(* Logix 5000 Program export IO_Mapping; software revision 30.00 *)

TYPE Std_DiscreteAlarm :   // ALARM RESET
STRUCT
   AckC : BOOL;   // ALARM ACKNOWLEDGE
   LatchA : BOOL;   // ALARM LATCH
   DetectS : BOOL;   // ALARM DETECT
   BitS : BOOL;   // ALARM MISCOMPARE
   InhibitC : BOOL;   // ALARM INHIBIT
   Tmr : TIMER;   // ALARM Timer
END_STRUCT
END_TYPE

TYPE VMAC_DATA_INTERNAL :
STRUCT
   VMACOK : BOOL;
   CommsOK : BOOL;
   KeyOK : BOOL;
   KsInUse : BOOL;
   KsPrimeInUse : BOOL;
   EntryStatus : INT;
   NodeID : DINT;
   DestinationID : DINT;
   Counter : LINT;
   LastCounter : LINT;
   KeyID : LINT;
   VMAC_KEY : DINT[8];
   VMAC_CALC : DINT[8];
   VMAC_INPUT : DINT[8];
   DATA_INPUT : DINT[1600];
   DATA_VERIFIED : DINT[1600];
   VMAC_CTRL : VMAC;
   KeyAlarm : Std_DiscreteAlarm;
   ReplayAlarm : Std_DiscreteAlarm;
   InvalidAlarm : Std_DiscreteAlarm;
   NodeAlarm : Std_DiscreteAlarm;
   DestinationAlarm : Std_DiscreteAlarm;
   L_LES : L_LES;
   L_EQU : L_EQU;
   CommsTimer : TIMER;
END_STRUCT
END_TYPE

TYPE VMAC_DATA_MSG :
STRUCT
   STATUS : CONNECTION_STATUS;
   DATA : DINT[100];
   LEN : DINT;
   ROUNDS : DINT;
   VMAC : DINT[8];
END_STRUCT
END_TYPE

ADD_ON_INSTRUCTION D_SHR   (* revision 1.0 20170524, vendor Kenneth A. Fischer *)
// DINT bit shift right of the 32-bit argument Inp_A by Inp_B bits with paddding by zeros on the right
// Revision note:
// Rev1.0: 20170524 - Initial Release
VAR_IN_OUT
   Inp_A : DINT; {required}   // 64-bit Integer to be right circular rotated
END_VAR
VAR_INPUT
   Inp_B : INT; {required}   // Number of bits to shift
END_VAR
VAR_IN_OUT
   Out : DINT; {required}   // Result
END_VAR
VAR
   BSR_Cntrl : CONTROL := (LEN := 32);
   ONS : BOOL;
   Source_Bit : BOOL;
   Wrk_InpA : DINT[2];
END_VAR

ROUTINE Logic   (* ladder *)
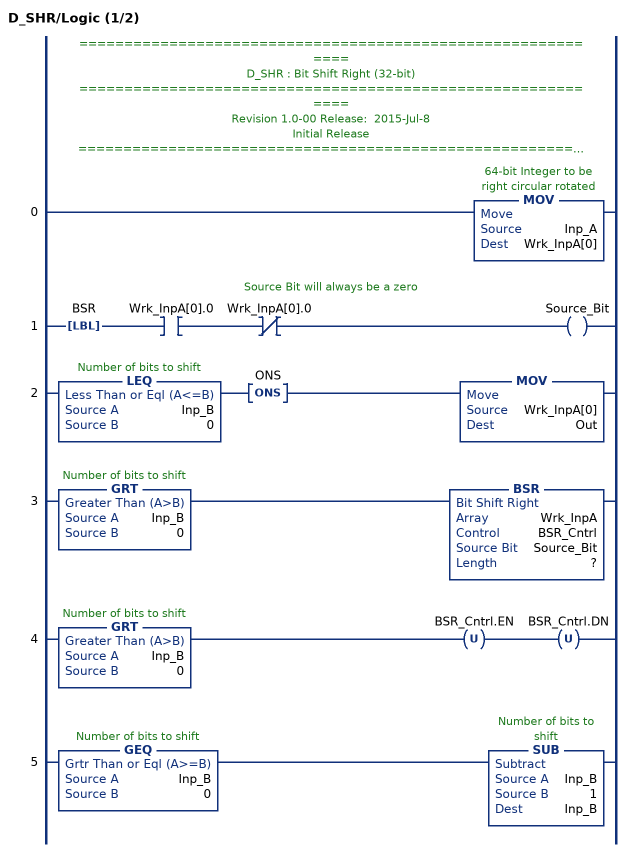
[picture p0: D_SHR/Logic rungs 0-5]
   // ============================================================
   // D_SHR : Bit Shift Right (32-bit)
   // ============================================================
   // Revision 1.0-00 Release:  2015-Jul-8
   // Initial Release
   // ============================================================
   // Performs a right bit shift of the 32-bit argument Inp_A by the
   // number of bits defined in the 16-bit argument Inp_B, with padding by zeros.
   0: MOV(Inp_A,Wrk_InpA[0]);
   // Source Bit will always be a zero
   1: LBL(BSR)XIC(Wrk_InpA[0].0)XIO(Wrk_InpA[0].0)OTE(Source_Bit);
   2: LEQ(Inp_B,0)ONS(ONS)MOV(Wrk_InpA[0],Out);
   3: GRT(Inp_B,0)BSR(Wrk_InpA,BSR_Cntrl,Source_Bit,?);
   4: GRT(Inp_B,0)OTU(BSR_Cntrl.EN)OTU(BSR_Cntrl.DN);
   5: GEQ(Inp_B,0)SUB(Inp_B,1,Inp_B);
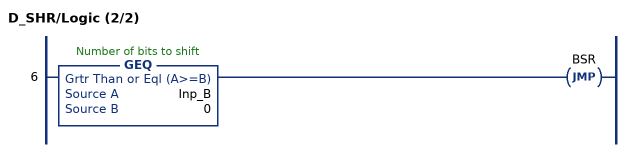
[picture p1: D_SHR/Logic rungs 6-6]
   6: GEQ(Inp_B,0)JMP(BSR);
END_ROUTINE
END_ADD_ON_INSTRUCTION

ADD_ON_INSTRUCTION D_SHL   (* revision 1.0 20170524, vendor Kenneth A. Fischer *)
// DINT bit shift left of the 32-bit argument Inp_A by Inp_B bits with paddding by zeros on the right
// Revision note:
// Rev1.0: 20170524 - Initial Release
VAR_IN_OUT
   Inp_A : DINT; {required}   // 64-bit Integer to be right circular rotated
END_VAR
VAR_INPUT
   Inp_B : INT; {required}   // Number of bits to shift
END_VAR
VAR_IN_OUT
   Out : DINT; {required}   // Result
END_VAR
VAR
   Wrk_InpA : DINT[2];
   Source_Bit : BOOL;
   ONS : BOOL;
   BSL_Cntrl : CONTROL := (LEN := 32);
END_VAR

ROUTINE Logic   (* ladder *)
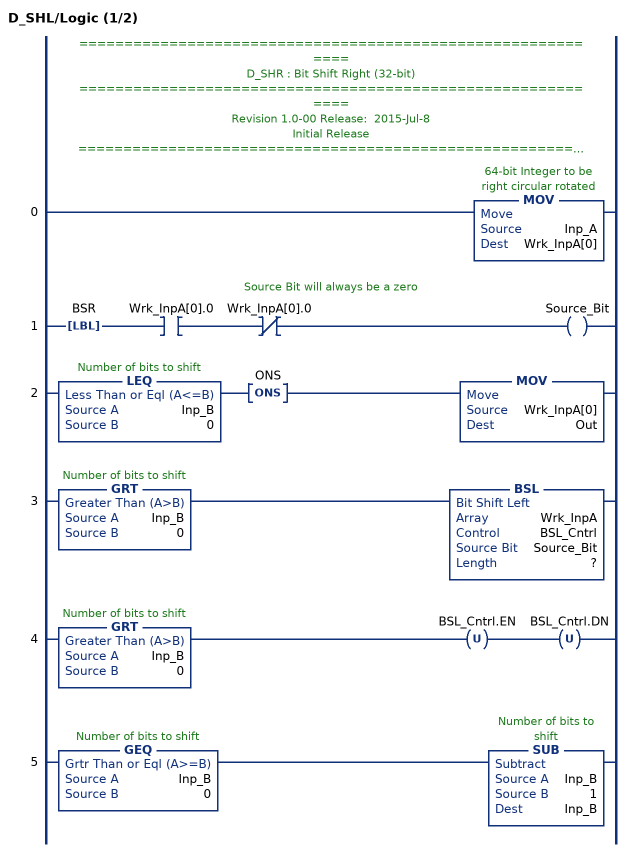
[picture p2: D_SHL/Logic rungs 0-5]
   // ============================================================
   // D_SHR : Bit Shift Right (32-bit)
   // ============================================================
   // Revision 1.0-00 Release:  2015-Jul-8
   // Initial Release
   // ============================================================
   // Performs a left bit shift of the 32-bit argument Inp_A by the
   // number of bits defined in the 16-bit argument Inp_B, with padding by zeros.
   0: MOV(Inp_A,Wrk_InpA[0]);
   // Source Bit will always be a zero
   1: LBL(BSR)XIC(Wrk_InpA[0].0)XIO(Wrk_InpA[0].0)OTE(Source_Bit);
   2: LEQ(Inp_B,0)ONS(ONS)MOV(Wrk_InpA[0],Out);
   3: GRT(Inp_B,0)BSL(Wrk_InpA,BSL_Cntrl,Source_Bit,?);
   4: GRT(Inp_B,0)OTU(BSL_Cntrl.EN)OTU(BSL_Cntrl.DN);
   5: GEQ(Inp_B,0)SUB(Inp_B,1,Inp_B);
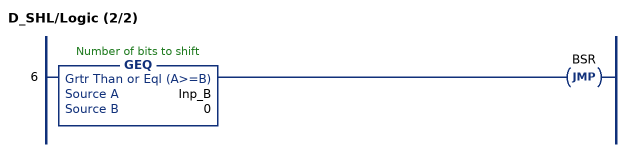
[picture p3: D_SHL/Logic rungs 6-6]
   6: GEQ(Inp_B,0)JMP(BSR);
END_ROUTINE
END_ADD_ON_INSTRUCTION

ADD_ON_INSTRUCTION B256_CtoE   (* revision 1.0 20170916, vendor Kenneth A. Fischer *)
// Convert 256-bit value using 22 12-bit pieces into 256-bit value using 32 8-bit pieces
// Revision note:
// Rev1.0: 20170916 - Initial Release
VAR_IN_OUT
   Inp_C : DINT[22]; {required}
   Out_E : DINT[32]; {required}
END_VAR
VAR
   i : INT;
   j : INT;
   TEMP1 : DINT;
   TEMP2 : DINT;
   D_SHL : D_SHL;
   D_SHR : D_SHR;
END_VAR

ROUTINE Logic   (* ladder *)
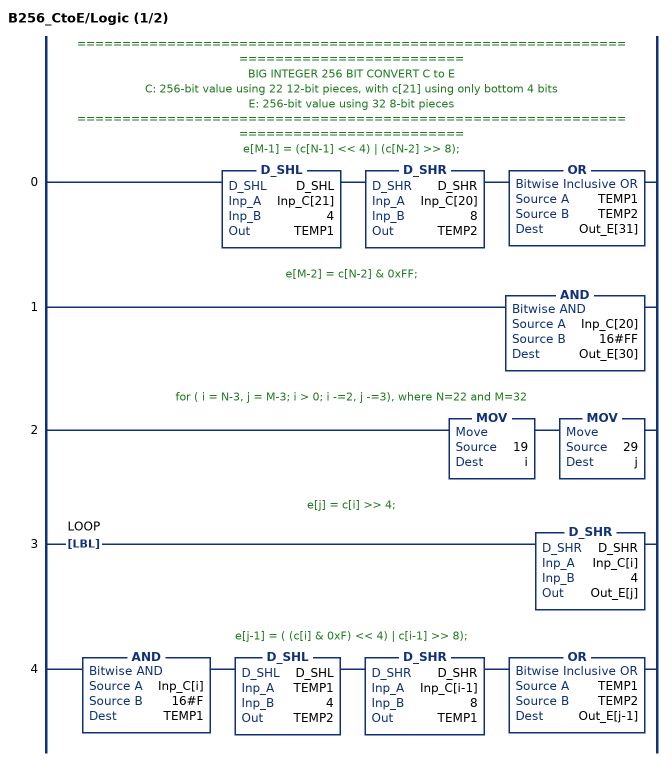
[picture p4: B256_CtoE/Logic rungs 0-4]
   // ======================================================================================
   // BIG INTEGER 256 BIT CONVERT C to E
   // C: 256-bit value using 22 12-bit pieces, with c[21] using only bottom 4 bits
   // E: 256-bit value using 32 8-bit pieces
   // ======================================================================================
   // e[M-1] = (c[N-1] << 4) | (c[N-2] >> 8);
   0: D_SHL(D_SHL,Inp_C[21],4,TEMP1)D_SHR(D_SHR,Inp_C[20],8,TEMP2)OR(TEMP1,TEMP2,Out_E[31]);
   // e[M-2] = c[N-2] & 0xFF;
   1: AND(Inp_C[20],16#FF,Out_E[30]);
   // for ( i = N-3, j = M-3; i > 0; i -=2, j -=3), where N=22 and M=32
   2: MOV(19,i)MOV(29,j);
   // e[j] = c[i] >> 4;
   3: LBL(LOOP)D_SHR(D_SHR,Inp_C[i],4,Out_E[j]);
   // e[j-1] = ( (c[i] & 0xF) << 4) | c[i-1] >> 8);
   4: AND(Inp_C[i],16#F,TEMP1)D_SHL(D_SHL,TEMP1,4,TEMP2)D_SHR(D_SHR,Inp_C[i-1],8,TEMP1)OR(TEMP1,TEMP2,Out_E[j-1]);
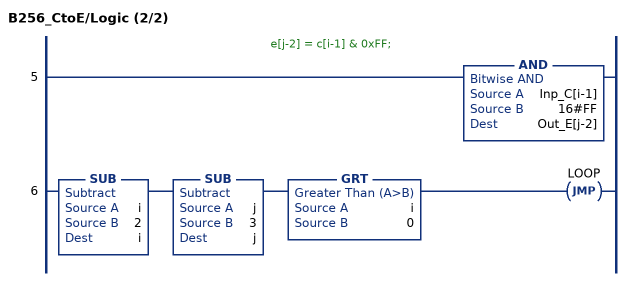
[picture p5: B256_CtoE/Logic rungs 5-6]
   // e[j-2] = c[i-1] & 0xFF;
   5: AND(Inp_C[i-1],16#FF,Out_E[j-2]);
   6: SUB(i,2,i)SUB(j,3,j)GRT(i,0)JMP(LOOP);
END_ROUTINE
END_ADD_ON_INSTRUCTION

ADD_ON_INSTRUCTION B256_StoC   (* revision 1.0 20170916, vendor Kenneth A. Fischer *)
// Convert 256-bit value using 64 hex string characters into 256-bit value using 22 12-bit pieces
// Revision note:
// Rev1.0: 20170916 - Initial Release
VAR_IN_OUT
   Inp_S : STRING; {required}
   Out_C : DINT[22]; {required}
END_VAR
VAR
   byte : DINT[3];
   D_SHL : D_SHL;
   i : INT;
   j : INT;
   k : DINT;
   temp : DINT;
END_VAR

ROUTINE Logic   (* ladder *)
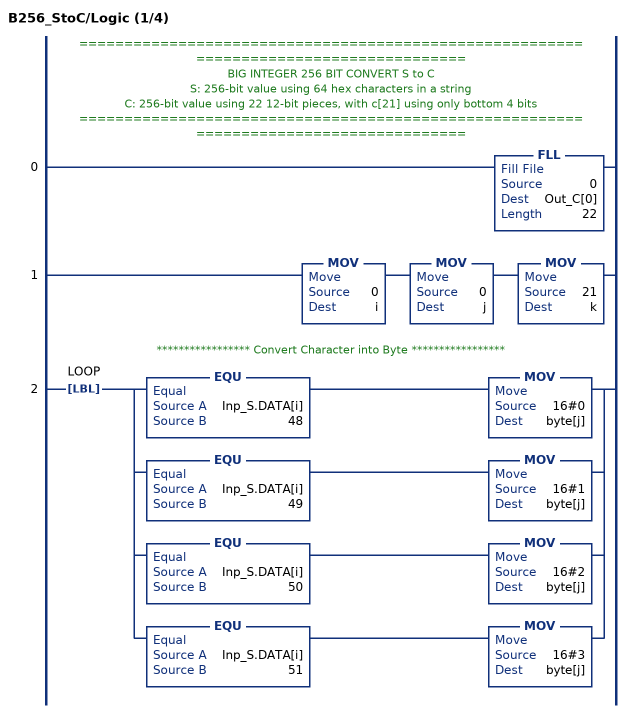
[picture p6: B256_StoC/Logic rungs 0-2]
   // ======================================================================================
   // BIG INTEGER 256 BIT CONVERT S to C
   // S: 256-bit value using 64 hex characters in a string
   // C: 256-bit value using 22 12-bit pieces, with c[21] using only bottom 4 bits
   // ======================================================================================
   0: FLL(0,Out_C[0],22);
   1: MOV(0,i)MOV(0,j)MOV(21,k);
   // ***************** Convert Character into Byte *****************
   2: LBL(LOOP)[EQU(Inp_S.DATA[i],48) MOV(16#0,byte[j]) ,EQU(Inp_S.DATA[i],49) MOV(16#1,byte[j]) ,EQU(Inp_S.DATA[i],50) MOV(16#2,byte[j]) ,EQU(Inp_S.DATA[i],51) MOV(16#3,byte[j]) ];
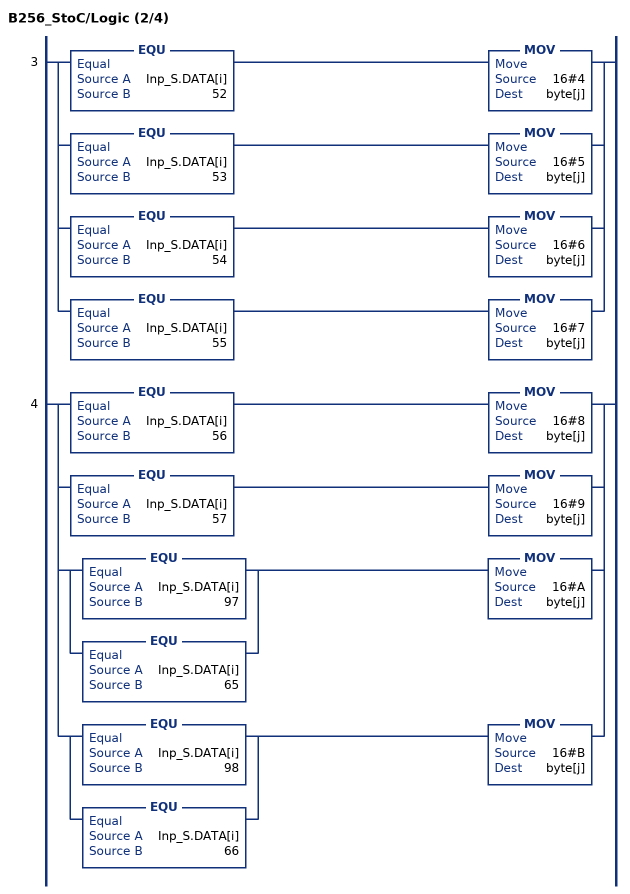
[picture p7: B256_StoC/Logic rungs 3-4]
   3: [EQU(Inp_S.DATA[i],52) MOV(16#4,byte[j]) ,EQU(Inp_S.DATA[i],53) MOV(16#5,byte[j]) ,EQU(Inp_S.DATA[i],54) MOV(16#6,byte[j]) ,EQU(Inp_S.DATA[i],55) MOV(16#7,byte[j]) ];
   4: [EQU(Inp_S.DATA[i],56) MOV(16#8,byte[j]) ,EQU(Inp_S.DATA[i],57) MOV(16#9,byte[j]) ,[EQU(Inp_S.DATA[i],97) ,EQU(Inp_S.DATA[i],65) ] MOV(16#A,byte[j]) ,[EQU(Inp_S.DATA[i],98) ,EQU(Inp_S.DATA[i],66) ] MOV(16#B,byte[j]) ];
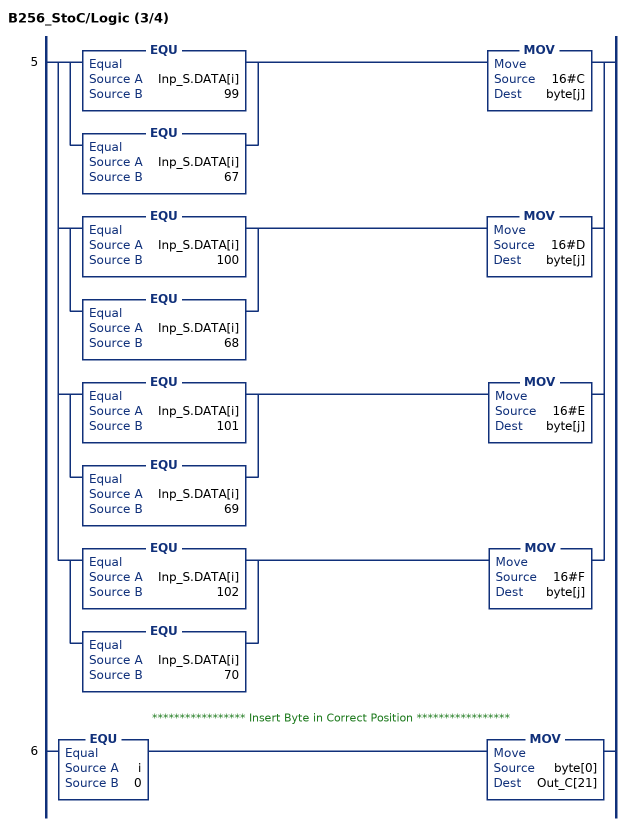
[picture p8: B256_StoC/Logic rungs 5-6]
   5: [[EQU(Inp_S.DATA[i],99) ,EQU(Inp_S.DATA[i],67) ] MOV(16#C,byte[j]) ,[EQU(Inp_S.DATA[i],100) ,EQU(Inp_S.DATA[i],68) ] MOV(16#D,byte[j]) ,[EQU(Inp_S.DATA[i],101) ,EQU(Inp_S.DATA[i],69) ] MOV(16#E,byte[j]) ,[EQU(Inp_S.DATA[i],102) ,EQU(Inp_S.DATA[i],70) ] MOV(16#F,byte[j]) ];
   // ***************** Insert Byte in Correct Position *****************
   6: EQU(i,0)MOV(byte[0],Out_C[21]);
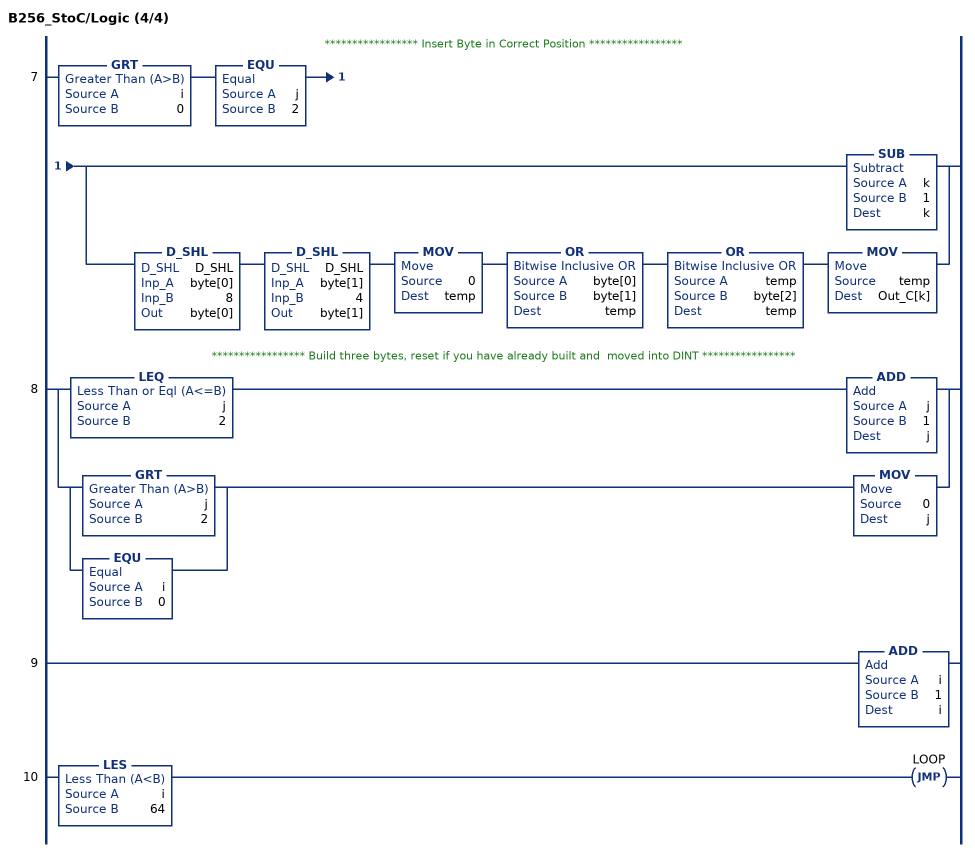
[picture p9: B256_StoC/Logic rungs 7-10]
   // ***************** Insert Byte in Correct Position *****************
   7: GRT(i,0)EQU(j,2)[SUB(k,1,k) ,D_SHL(D_SHL,byte[0],8,byte[0]) D_SHL(D_SHL,byte[1],4,byte[1]) MOV(0,temp) OR(byte[0],byte[1],temp) OR(temp,byte[2],temp) MOV(temp,Out_C[k]) ];
   // ***************** Build three bytes, reset if you have already built and  moved into DINT *****************
   8: [LEQ(j,2) ADD(j,1,j) ,[GRT(j,2) ,EQU(i,0) ] MOV(0,j) ];
   9: ADD(i,1,i);
   10: LES(i,64)JMP(LOOP);
END_ROUTINE
END_ADD_ON_INSTRUCTION

ADD_ON_INSTRUCTION L_INC   (* revision 1.0 00 Release, vendor Rockwell Automation *)
// Increment (64-bit)
// Revision note:
// Initial Release
// Help:
// This instruction increments the input 64-bit integer, returning its value plus 1.
VAR_IN_OUT
   Inp : LINT; {required}   // Input
   Out : LINT; {required}   // Output = Input + 1
END_VAR
VAR
   Wrk : DINT[2];   // Working pair of 32-bit integers (DINTs)
   Wrk_LoOvflw : BOOL;   // Low-order 32-bit overflow (without minor fault)
   Wrk_HiOvflw : BOOL;   // High-order 32-bit overflow (without minor fault)
END_VAR

ROUTINE Logic   (* ladder *)
// Output the value of the input plus 1
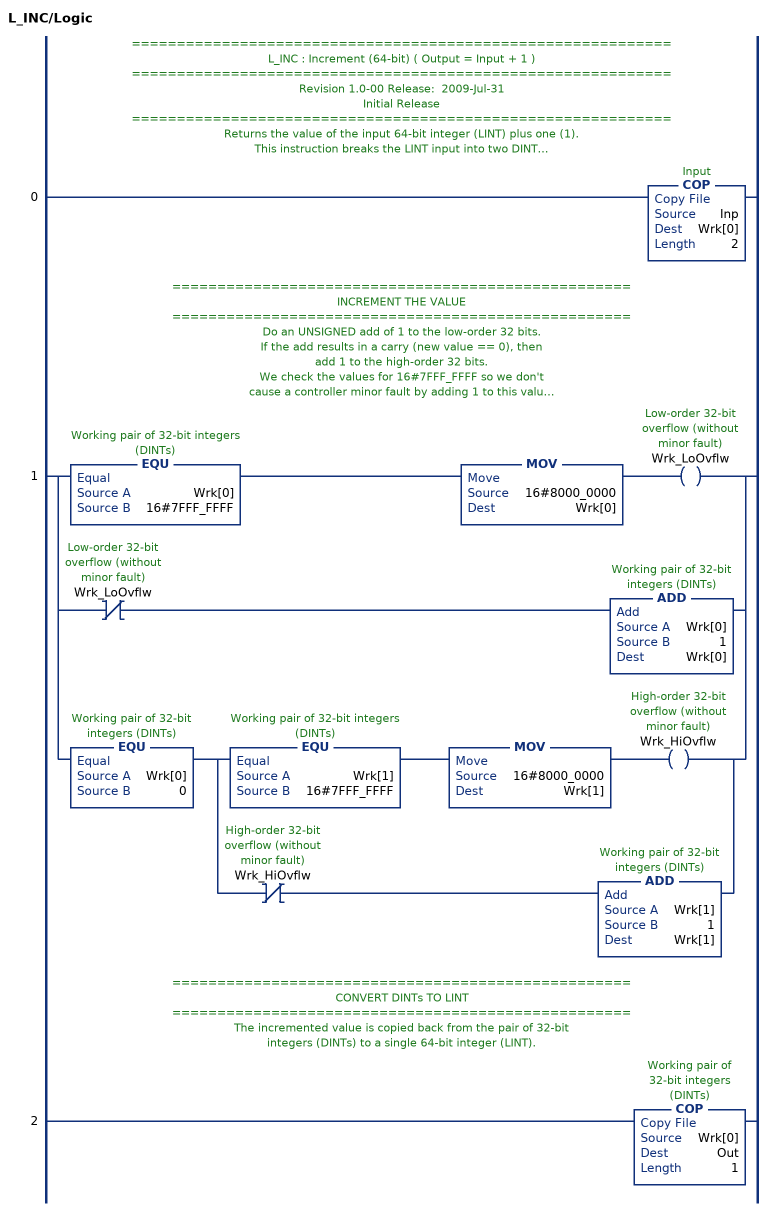
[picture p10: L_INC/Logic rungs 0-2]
   // ============================================================
   // L_INC : Increment (64-bit) ( Output = Input + 1 )
   // ============================================================
   // Revision 1.0-00 Release:  2009-Jul-31
   // Initial Release
   // ============================================================
   // Returns the value of the input 64-bit integer (LINT) plus one (1).
   // This instruction breaks the LINT input into two DINTs
   // (32-bit signed each) to do the math.
   // ===================================================
   // CONVERT LINT TO DINTs
   // ===================================================
   // This COPy takes the input LINT and breaks it into a pair of DINTs.
   0: COP(Inp,Wrk[0],2);
   // ===================================================
   // INCREMENT THE VALUE
   // ===================================================
   // Do an UNSIGNED add of 1 to the low-order 32 bits.
   // If the add results in a carry (new value == 0), then
   // add 1 to the high-order 32 bits.
   // We check the values for 16#7FFF_FFFF so we don't
   // cause a controller minor fault by adding 1 to this value
   // (resulting in a signed overflow to negative).
   1: [EQU(Wrk[0],16#7FFF_FFFF) MOV(16#8000_0000,Wrk[0]) OTE(Wrk_LoOvflw) ,XIO(Wrk_LoOvflw) ADD(Wrk[0],1,Wrk[0]) ,EQU(Wrk[0],0) [EQU(Wrk[1],16#7FFF_FFFF) MOV(16#8000_0000,Wrk[1]) OTE(Wrk_HiOvflw) ,XIO(Wrk_HiOvflw) ADD(Wrk[1],1,Wrk[1]) ] ];
   // ===================================================
   // CONVERT DINTs TO LINT
   // ===================================================
   // The incremented value is copied back from the pair of 32-bit
   // integers (DINTs) to a single 64-bit integer (LINT).
   2: COP(Wrk[0],Out,1);
END_ROUTINE
END_ADD_ON_INSTRUCTION

ADD_ON_INSTRUCTION B256_EtoDINT   (* revision 1.0 20170916, vendor Kenneth A. Fischer *)
// Convert 256-bit value using 32 8-bit pieces into 256-bit value using 8 32-bit pieces
// Revision note:
// Rev1.0: 20170916 - Initial Release
VAR_IN_OUT
   Inp_E : DINT[32]; {required}
   Out_DINT : DINT[8]; {required}
END_VAR
VAR
   D_SHL : D_SHL;
   i : INT;
   j : INT;
   TEMP : DINT;
END_VAR

ROUTINE Logic   (* ladder *)
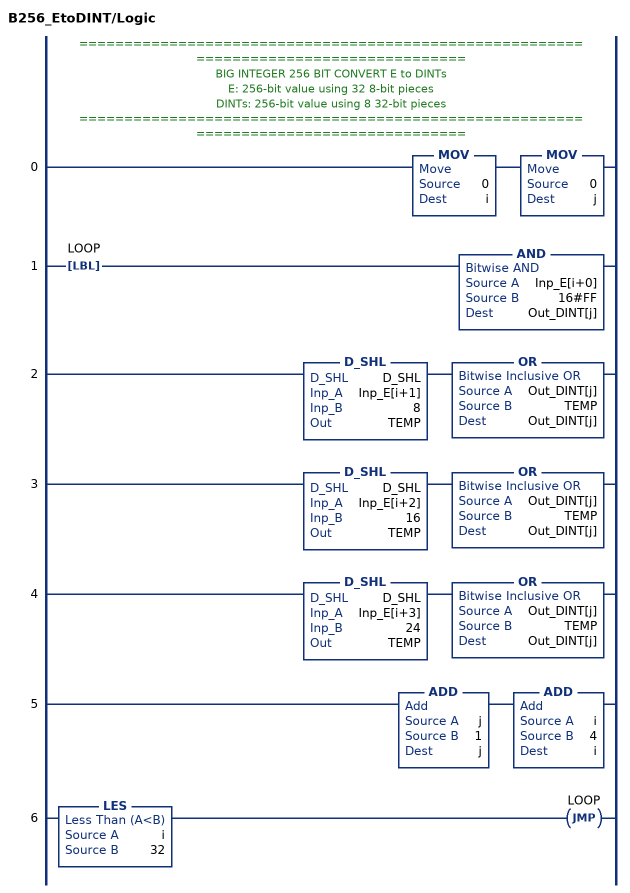
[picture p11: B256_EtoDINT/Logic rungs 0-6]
   // ======================================================================================
   // BIG INTEGER 256 BIT CONVERT E to DINTs
   // E: 256-bit value using 32 8-bit pieces
   // DINTs: 256-bit value using 8 32-bit pieces
   // ======================================================================================
   0: MOV(0,i)MOV(0,j);
   1: LBL(LOOP)AND(Inp_E[i+0],16#FF,Out_DINT[j]);
   2: D_SHL(D_SHL,Inp_E[i+1],8,TEMP)OR(Out_DINT[j],TEMP,Out_DINT[j]);
   3: D_SHL(D_SHL,Inp_E[i+2],16,TEMP)OR(Out_DINT[j],TEMP,Out_DINT[j]);
   4: D_SHL(D_SHL,Inp_E[i+3],24,TEMP)OR(Out_DINT[j],TEMP,Out_DINT[j]);
   5: ADD(j,1,j)ADD(i,4,i);
   6: LES(i,32)JMP(LOOP);
END_ROUTINE
END_ADD_ON_INSTRUCTION

ADD_ON_INSTRUCTION D_ROTR   (* revision 1.0 20170524, vendor Kenneth A. Fischer *)
// DINT circular right shift (rotation) of the 32-bit argument Inp_A by Inp_B bits
// Revision note:
// Rev1.0: 20170524 - Initial Release
VAR_IN_OUT
   Inp_A : DINT; {required}   // 64-bit Integer to be right circular rotated
END_VAR
VAR_INPUT
   Inp_B : INT; {required}   // Number of Inp_A bit rotations
END_VAR
VAR_IN_OUT
   Out : DINT; {required}   // Result
END_VAR
VAR
   Wrk_InpA : DINT[2];
   BSR_Cntrl : CONTROL := (LEN := 32);
   Source_Bit : BOOL;
   ONS : BOOL;
END_VAR

ROUTINE Logic   (* ladder *)
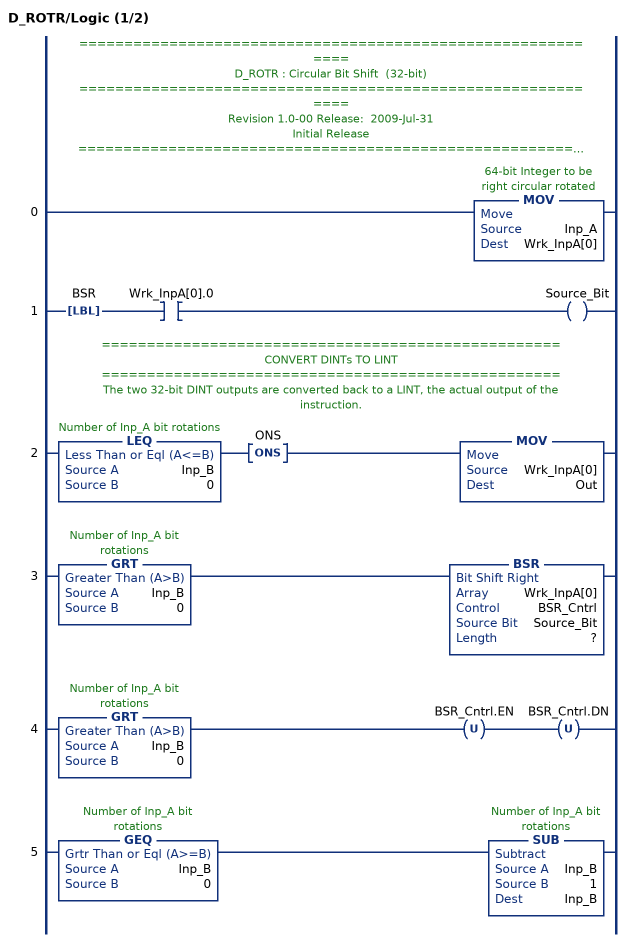
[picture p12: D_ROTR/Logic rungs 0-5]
   // ============================================================
   // D_ROTR : Circular Bit Shift  (32-bit)
   // ============================================================
   // Revision 1.0-00 Release:  2009-Jul-31
   // Initial Release
   // ============================================================
   // Performs a circular right shift rotation of the 32-bit argument Inp_A by the
   // number of bits defined in the 16-bit argument Inp_B.
   0: MOV(Inp_A,Wrk_InpA[0]);
   1: LBL(BSR)XIC(Wrk_InpA[0].0)OTE(Source_Bit);
   // ===================================================
   // CONVERT DINTs TO LINT
   // ===================================================
   // The two 32-bit DINT outputs are converted back to a LINT, the actual output of the instruction.
   2: LEQ(Inp_B,0)ONS(ONS)MOV(Wrk_InpA[0],Out);
   3: GRT(Inp_B,0)BSR(Wrk_InpA[0],BSR_Cntrl,Source_Bit,?);
   4: GRT(Inp_B,0)OTU(BSR_Cntrl.EN)OTU(BSR_Cntrl.DN);
   5: GEQ(Inp_B,0)SUB(Inp_B,1,Inp_B);
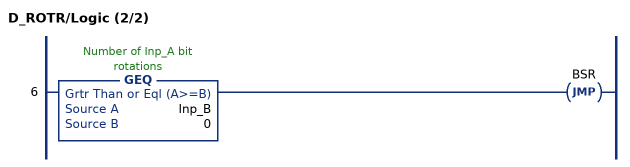
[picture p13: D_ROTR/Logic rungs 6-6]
   6: GEQ(Inp_B,0)JMP(BSR);
END_ROUTINE
END_ADD_ON_INSTRUCTION

ADD_ON_INSTRUCTION VMAC   (* revision 1.0 20170524, vendor Kenneth A. Fischer *)
// Variable Round MAC
// Revision note:
// Rev1.0: 20170524 - Initial Release
VAR_IN_OUT
   Inp_KEY : DINT[8]; {required}
   Inp_MSG : DINT[500]; {required}
END_VAR
VAR_INPUT
   Inp_LEN : DINT; {required}   // LENGTH INPUT OF MSG IN NUMBER OF DINTS
   Inp_ROUNDS : DINT; {required}
END_VAR
VAR_IN_OUT
   Out_VMAC : DINT[8]; {required}
        [0]   // HashBuffer_A
        [1]   // HashBuffer_B
        [2]   // HashBuffer_C
        [3]   // HashBuffer_D
        [4]   // HashBuffer_E
        [5]   // HashBuffer_F
        [6]   // HashBuffer_G
        [7]   // HashBuffer_H
END_VAR
VAR
   MajFunc : DINT;
   HashBuffer_H : DINT;
   HashBuffer_G : DINT;
   HashBuffer_F : DINT;
   HashBuffer_E : DINT;
   HashBuffer_D : DINT;
   HashBuffer_C : DINT;
   HashBuffer_B : DINT;
   HashBuffer_A : DINT;
   W : DINT[64];   // MESSAGE SCHEDULE
   tmp : DINT[20];
   T2 : DINT;
   T1 : DINT;
   t : INT;
   M : INT;   // MESSAGE INCREMENTS
   SigmaE : DINT;
   SigmaA : DINT;
   Sigma1 : DINT;
   Sigma0 : DINT;
   i : INT;
   x : INT;
   HashBufferInput_H : DINT;
   HashBufferInput_G : DINT;
   HashBufferInput_F : DINT;
   HashBufferInput_E : DINT;
   HashBufferInput_D : DINT;
   HashBufferInput_C : DINT;
   HashBufferInput_B : DINT;
   HashBufferInput_A : DINT;
   CondFunc : DINT;
   K : DINT[64];
   LENGTH_BITS : DINT;   // LENGTH OF MSG IN BITS
   LENGTH_MODULO : DINT;
   NUM_PADDING_BITS : DINT;   // NUMBER OF BITS NEEDED FOR PADDING
   NUM_PADDING_DINTS : DINT;   // NUMBER OF DINTS NEEDED FOR PADDING
   PADDING_COUNTER : DINT;
   TOTAL_MSG_LENGTH_MINUS_16 : DINT;
   D_ROTR : D_ROTR;
   D_SHR : D_SHR;
   ROUNDS : DINT;
   n : INT;
   KeyIndex : DINT;
   RotationIndex : DINT;
   IndexedKey : DINT;
END_VAR

ROUTINE Logic   (* ladder *)
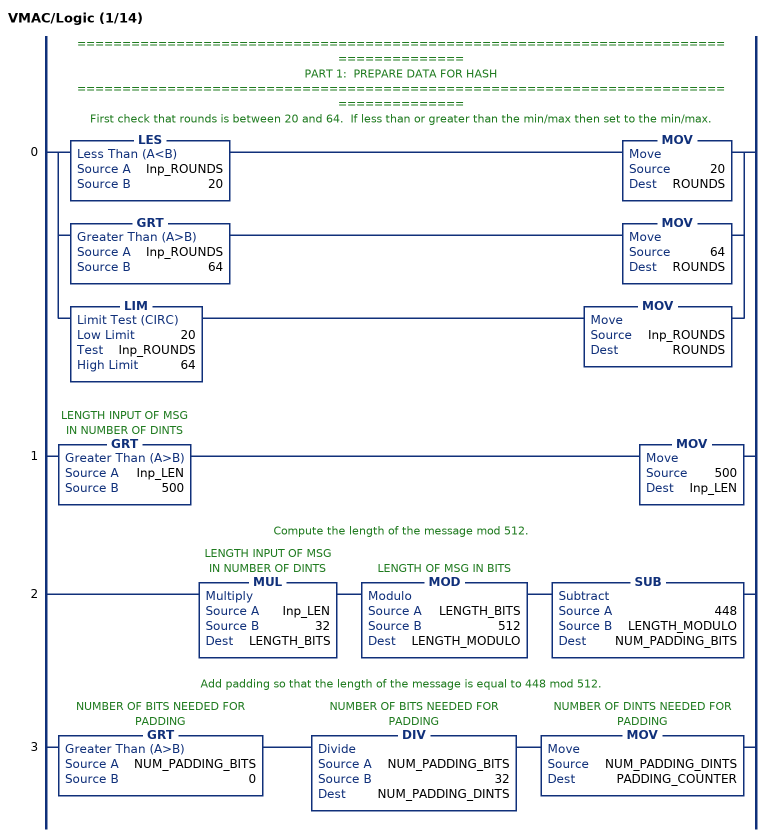
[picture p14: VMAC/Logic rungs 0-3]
   // ======================================================================================
   // PART 1:  PREPARE DATA FOR HASH
   // ======================================================================================
   // First check that rounds is between 20 and 64.  If less than or greater than the min/max then set to the min/max.
   0: [LES(Inp_ROUNDS,20) MOV(20,ROUNDS) ,GRT(Inp_ROUNDS,64) MOV(64,ROUNDS) ,LIM(20,Inp_ROUNDS,64) MOV(Inp_ROUNDS,ROUNDS) ];
   1: GRT(Inp_LEN,500)MOV(500,Inp_LEN);
   // Compute the length of the message mod 512.
   2: MUL(Inp_LEN,32,LENGTH_BITS)MOD(LENGTH_BITS,512,LENGTH_MODULO)SUB(448,LENGTH_MODULO,NUM_PADDING_BITS);
   // Add padding so that the length of the message is equal to 448 mod 512.
   3: GRT(NUM_PADDING_BITS,0)DIV(NUM_PADDING_BITS,32,NUM_PADDING_DINTS)MOV(NUM_PADDING_DINTS,PADDING_COUNTER);
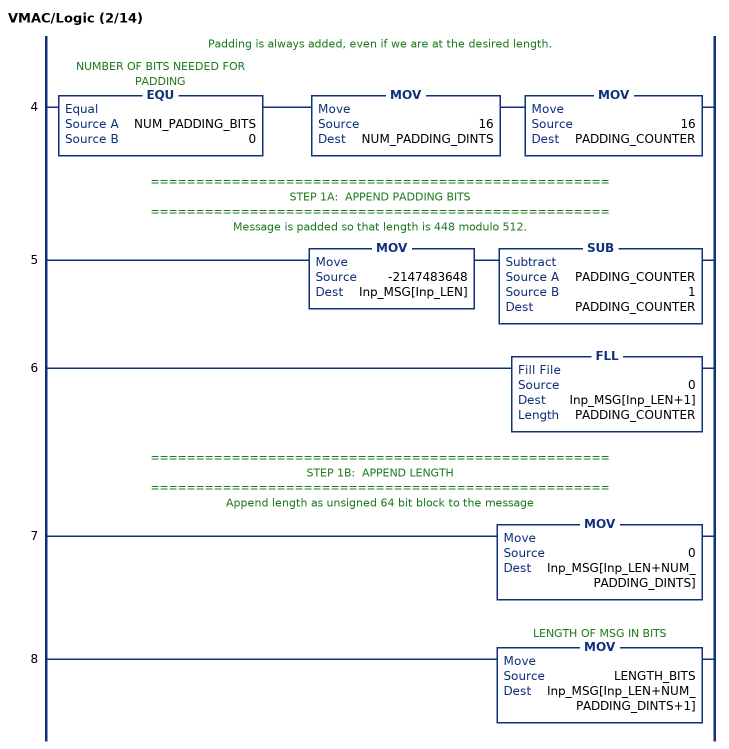
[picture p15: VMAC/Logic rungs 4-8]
   // Padding is always added, even if we are at the desired length.
   4: EQU(NUM_PADDING_BITS,0)MOV(16,NUM_PADDING_DINTS)MOV(16,PADDING_COUNTER);
   // ===================================================
   // STEP 1A:  APPEND PADDING BITS
   // ===================================================
   // Message is padded so that length is 448 modulo 512.
   5: MOV(-2147483648,Inp_MSG[Inp_LEN])SUB(PADDING_COUNTER,1,PADDING_COUNTER);
   6: FLL(0,Inp_MSG[Inp_LEN+1],PADDING_COUNTER);
   // ===================================================
   // STEP 1B:  APPEND LENGTH
   // ===================================================
   // Append length as unsigned 64 bit block to the message
   7: MOV(0,Inp_MSG[Inp_LEN+NUM_PADDING_DINTS]);
   8: MOV(LENGTH_BITS,Inp_MSG[Inp_LEN+NUM_PADDING_DINTS+1]);
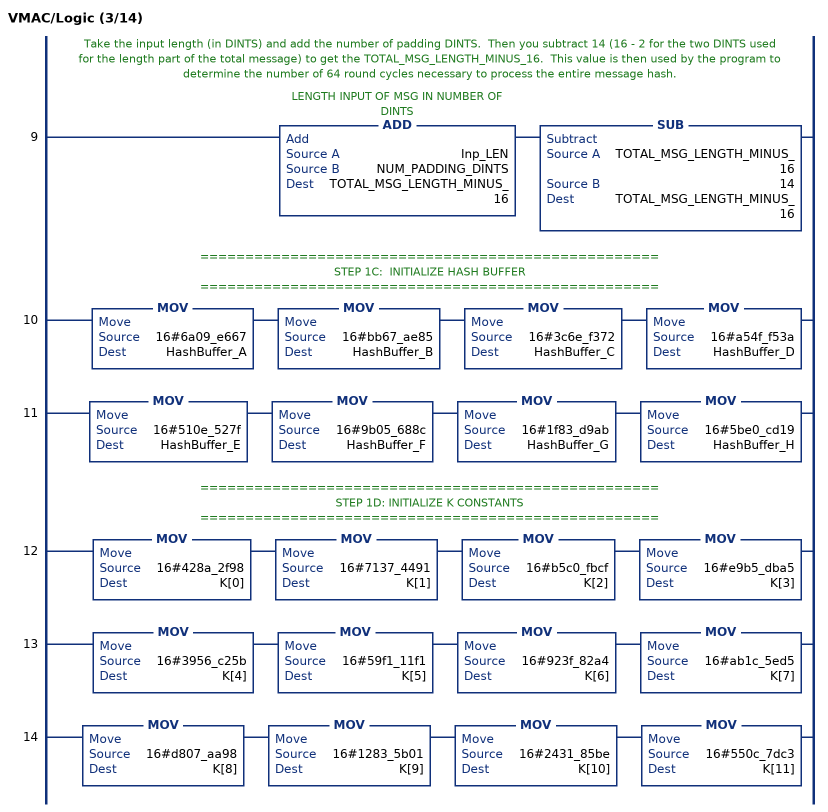
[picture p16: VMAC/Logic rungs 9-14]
   // Take the input length (in DINTS) and add the number of padding DINTS.  Then you subtract 14 (16 - 2 for the two DINTS used for the length part of the total message) to get the TOTAL_MSG_LENGTH_MINUS_16.  This value is then used by the program to determine the number of 64 round cycles necessary to process the entire message hash.
   9: ADD(Inp_LEN,NUM_PADDING_DINTS,TOTAL_MSG_LENGTH_MINUS_16)SUB(TOTAL_MSG_LENGTH_MINUS_16,14,TOTAL_MSG_LENGTH_MINUS_16);
   // ===================================================
   // STEP 1C:  INITIALIZE HASH BUFFER
   // ===================================================
   10: MOV(16#6a09_e667,HashBuffer_A)MOV(16#bb67_ae85,HashBuffer_B)MOV(16#3c6e_f372,HashBuffer_C)MOV(16#a54f_f53a,HashBuffer_D);
   11: MOV(16#510e_527f,HashBuffer_E)MOV(16#9b05_688c,HashBuffer_F)MOV(16#1f83_d9ab,HashBuffer_G)MOV(16#5be0_cd19,HashBuffer_H);
   // ===================================================
   // STEP 1D: INITIALIZE K CONSTANTS
   // ===================================================
   12: MOV(16#428a_2f98,K[0])MOV(16#7137_4491,K[1])MOV(16#b5c0_fbcf,K[2])MOV(16#e9b5_dba5,K[3]);
   13: MOV(16#3956_c25b,K[4])MOV(16#59f1_11f1,K[5])MOV(16#923f_82a4,K[6])MOV(16#ab1c_5ed5,K[7]);
   14: MOV(16#d807_aa98,K[8])MOV(16#1283_5b01,K[9])MOV(16#2431_85be,K[10])MOV(16#550c_7dc3,K[11]);
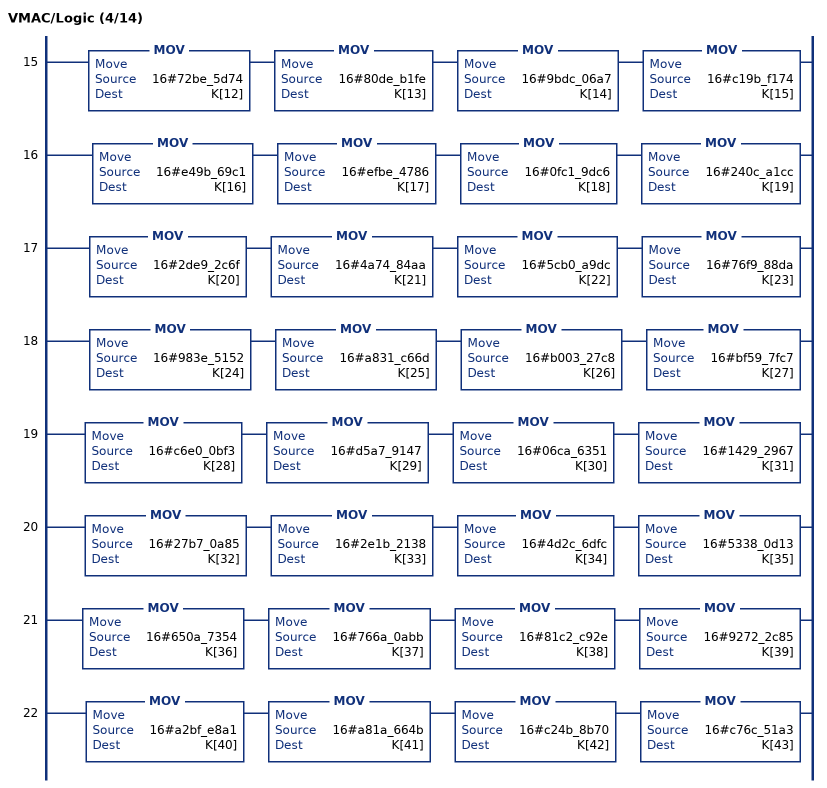
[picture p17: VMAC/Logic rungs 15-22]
   15: MOV(16#72be_5d74,K[12])MOV(16#80de_b1fe,K[13])MOV(16#9bdc_06a7,K[14])MOV(16#c19b_f174,K[15]);
   16: MOV(16#e49b_69c1,K[16])MOV(16#efbe_4786,K[17])MOV(16#0fc1_9dc6,K[18])MOV(16#240c_a1cc,K[19]);
   17: MOV(16#2de9_2c6f,K[20])MOV(16#4a74_84aa,K[21])MOV(16#5cb0_a9dc,K[22])MOV(16#76f9_88da,K[23]);
   18: MOV(16#983e_5152,K[24])MOV(16#a831_c66d,K[25])MOV(16#b003_27c8,K[26])MOV(16#bf59_7fc7,K[27]);
   19: MOV(16#c6e0_0bf3,K[28])MOV(16#d5a7_9147,K[29])MOV(16#06ca_6351,K[30])MOV(16#1429_2967,K[31]);
   20: MOV(16#27b7_0a85,K[32])MOV(16#2e1b_2138,K[33])MOV(16#4d2c_6dfc,K[34])MOV(16#5338_0d13,K[35]);
   21: MOV(16#650a_7354,K[36])MOV(16#766a_0abb,K[37])MOV(16#81c2_c92e,K[38])MOV(16#9272_2c85,K[39]);
   22: MOV(16#a2bf_e8a1,K[40])MOV(16#a81a_664b,K[41])MOV(16#c24b_8b70,K[42])MOV(16#c76c_51a3,K[43]);
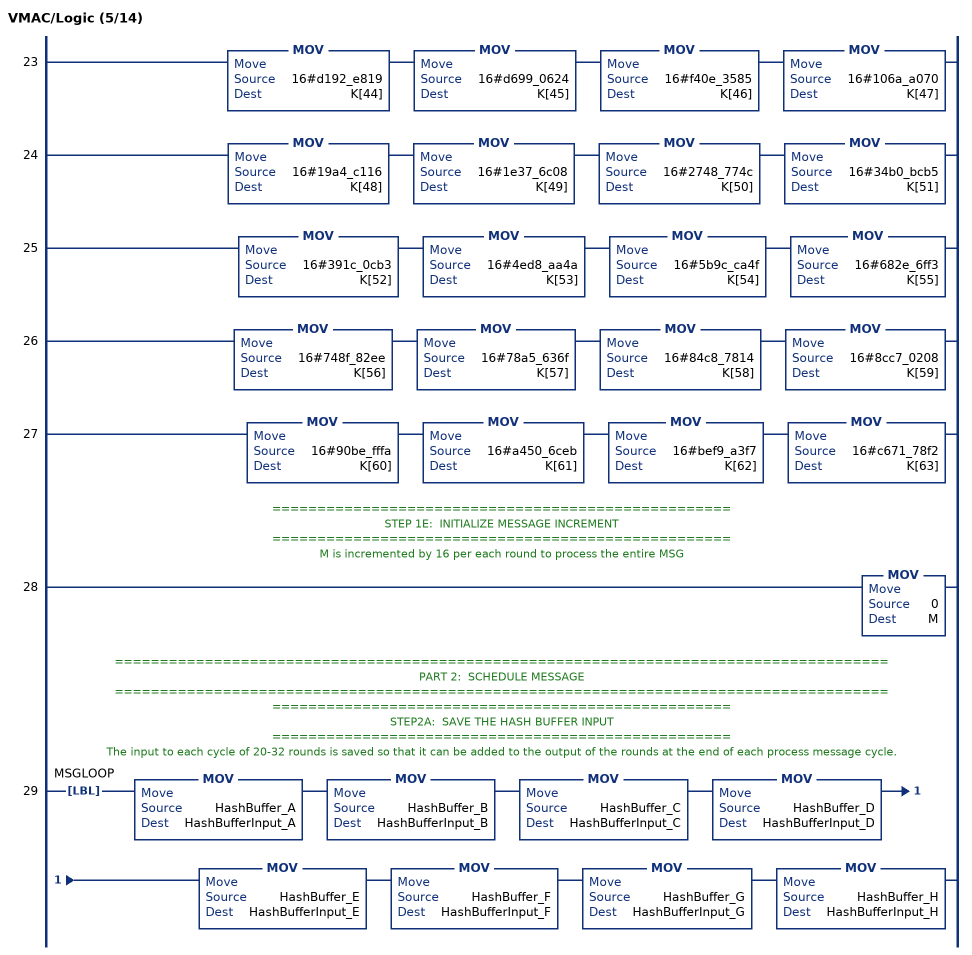
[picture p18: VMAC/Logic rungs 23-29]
   23: MOV(16#d192_e819,K[44])MOV(16#d699_0624,K[45])MOV(16#f40e_3585,K[46])MOV(16#106a_a070,K[47]);
   24: MOV(16#19a4_c116,K[48])MOV(16#1e37_6c08,K[49])MOV(16#2748_774c,K[50])MOV(16#34b0_bcb5,K[51]);
   25: MOV(16#391c_0cb3,K[52])MOV(16#4ed8_aa4a,K[53])MOV(16#5b9c_ca4f,K[54])MOV(16#682e_6ff3,K[55]);
   26: MOV(16#748f_82ee,K[56])MOV(16#78a5_636f,K[57])MOV(16#84c8_7814,K[58])MOV(16#8cc7_0208,K[59]);
   27: MOV(16#90be_fffa,K[60])MOV(16#a450_6ceb,K[61])MOV(16#bef9_a3f7,K[62])MOV(16#c671_78f2,K[63]);
   // ===================================================
   // STEP 1E:  INITIALIZE MESSAGE INCREMENT
   // ===================================================
   // M is incremented by 16 per each round to process the entire MSG
   28: MOV(0,M);
   // ======================================================================================
   // PART 2:  SCHEDULE MESSAGE
   // ======================================================================================
   // ===================================================
   // STEP2A:  SAVE THE HASH BUFFER INPUT
   // ===================================================
   // The input to each cycle of 20-32 rounds is saved so that it can be added to the output of the rounds at the end of each process message cycle.
   29: LBL(MSGLOOP)MOV(HashBuffer_A,HashBufferInput_A)MOV(HashBuffer_B,HashBufferInput_B)MOV(HashBuffer_C,HashBufferInput_C)MOV(HashBuffer_D,HashBufferInput_D)MOV(HashBuffer_E,HashBufferInput_E)MOV(HashBuffer_F,HashBufferInput_F)MOV(HashBuffer_G,HashBufferInput_G)MOV(HashBuffer_H,HashBufferInput_H);
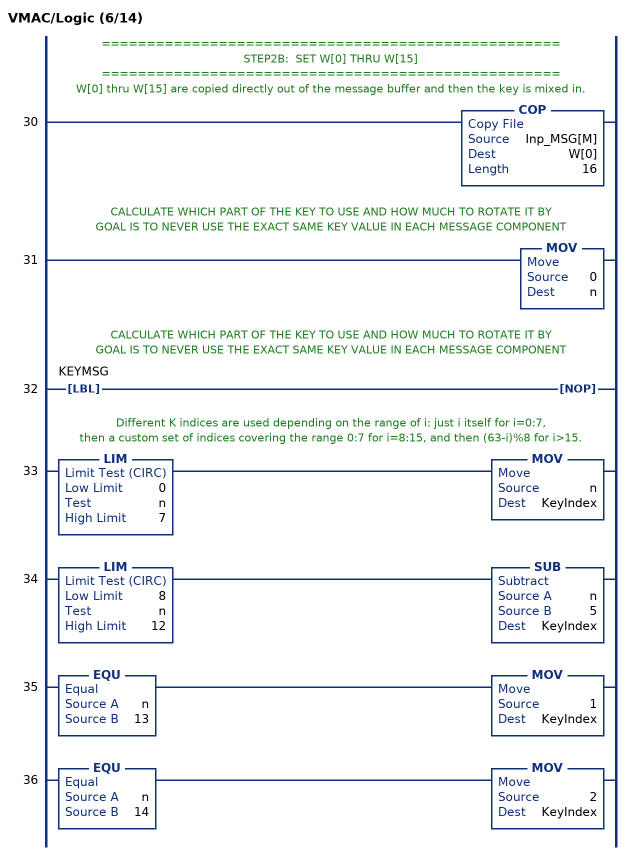
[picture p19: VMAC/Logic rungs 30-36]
   // ===================================================
   // STEP2B:  SET W[0] THRU W[15]
   // ===================================================
   // W[0] thru W[15] are copied directly out of the message buffer and then the key is mixed in.
   30: COP(Inp_MSG[M],W[0],16);
   // CALCULATE WHICH PART OF THE KEY TO USE AND HOW MUCH TO ROTATE IT BY
   // GOAL IS TO NEVER USE THE EXACT SAME KEY VALUE IN EACH MESSAGE COMPONENT
   31: MOV(0,n);
   // CALCULATE WHICH PART OF THE KEY TO USE AND HOW MUCH TO ROTATE IT BY
   // GOAL IS TO NEVER USE THE EXACT SAME KEY VALUE IN EACH MESSAGE COMPONENT
   32: LBL(KEYMSG)NOP();
   // Different K indices are used depending on the range of i: just i itself for i=0:7,
   // then a custom set of indices covering the range 0:7 for i=8:15, and then (63-i)%8 for i>15.
   33: LIM(0,n,7)MOV(n,KeyIndex);
   34: LIM(8,n,12)SUB(n,5,KeyIndex);
   35: EQU(n,13)MOV(1,KeyIndex);
   36: EQU(n,14)MOV(2,KeyIndex);
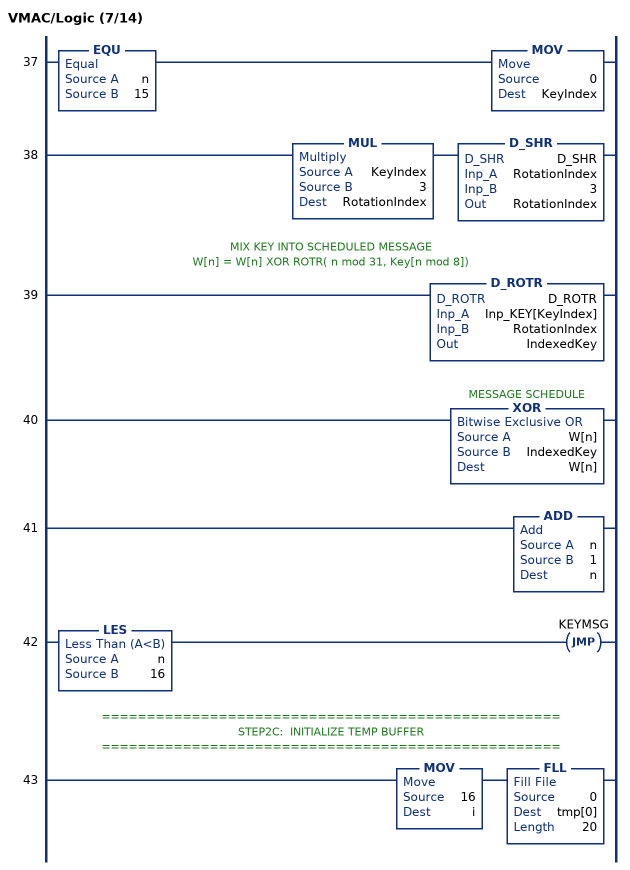
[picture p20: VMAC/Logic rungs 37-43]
   37: EQU(n,15)MOV(0,KeyIndex);
   38: MUL(KeyIndex,3,RotationIndex)D_SHR(D_SHR,RotationIndex,3,RotationIndex);
   // MIX KEY INTO SCHEDULED MESSAGE
   // W[n] = W[n] XOR ROTR( n mod 31, Key[n mod 8])
   39: D_ROTR(D_ROTR,Inp_KEY[KeyIndex],RotationIndex,IndexedKey);
   40: XOR(W[n],IndexedKey,W[n]);
   41: ADD(n,1,n);
   42: LES(n,16)JMP(KEYMSG);
   // ===================================================
   // STEP2C:  INITIALIZE TEMP BUFFER
   // ===================================================
   43: MOV(16,i)FLL(0,tmp[0],20);
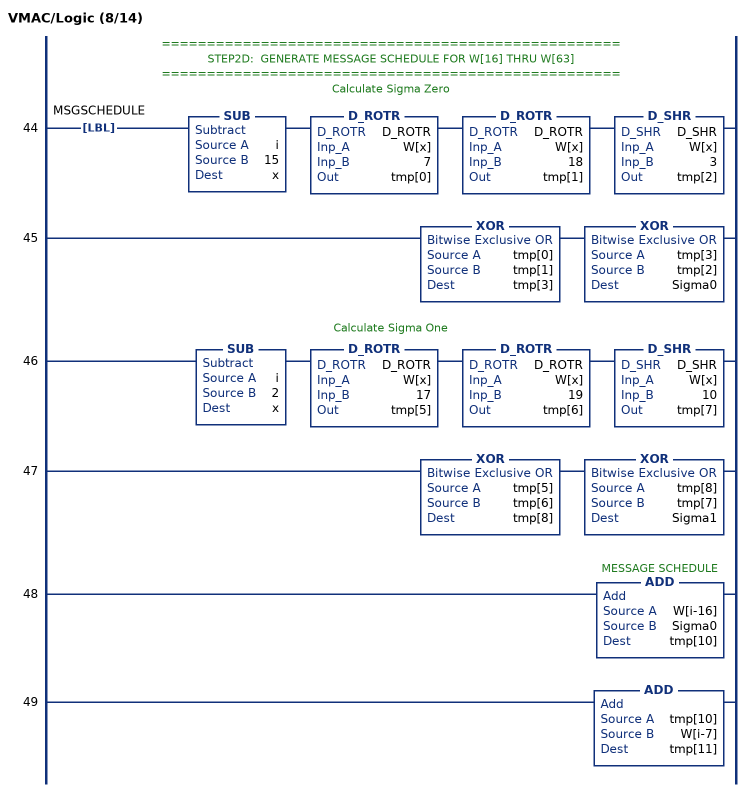
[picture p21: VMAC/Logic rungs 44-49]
   // ===================================================
   // STEP2D:  GENERATE MESSAGE SCHEDULE FOR W[16] THRU W[63]
   // ===================================================
   // Calculate Sigma Zero
   44: LBL(MSGSCHEDULE)SUB(i,15,x)D_ROTR(D_ROTR,W[x],7,tmp[0])D_ROTR(D_ROTR,W[x],18,tmp[1])D_SHR(D_SHR,W[x],3,tmp[2]);
   45: XOR(tmp[0],tmp[1],tmp[3])XOR(tmp[3],tmp[2],Sigma0);
   // Calculate Sigma One
   46: SUB(i,2,x)D_ROTR(D_ROTR,W[x],17,tmp[5])D_ROTR(D_ROTR,W[x],19,tmp[6])D_SHR(D_SHR,W[x],10,tmp[7]);
   47: XOR(tmp[5],tmp[6],tmp[8])XOR(tmp[8],tmp[7],Sigma1);
   48: ADD(W[i-16],Sigma0,tmp[10]);
   49: ADD(tmp[10],W[i-7],tmp[11]);
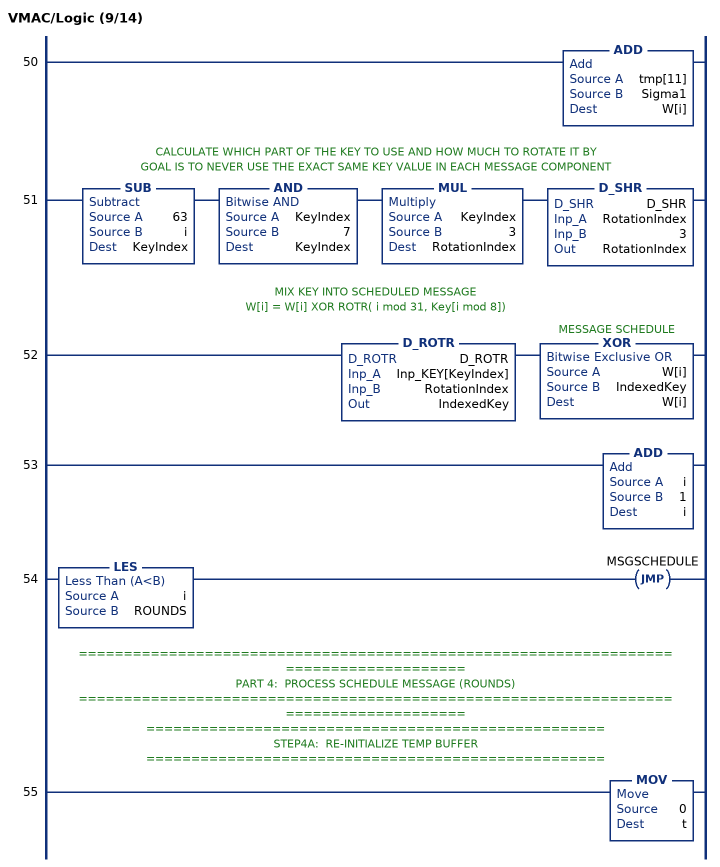
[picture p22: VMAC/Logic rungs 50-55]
   50: ADD(tmp[11],Sigma1,W[i]);
   // CALCULATE WHICH PART OF THE KEY TO USE AND HOW MUCH TO ROTATE IT BY
   // GOAL IS TO NEVER USE THE EXACT SAME KEY VALUE IN EACH MESSAGE COMPONENT
   51: SUB(63,i,KeyIndex)AND(KeyIndex,7,KeyIndex)MUL(KeyIndex,3,RotationIndex)D_SHR(D_SHR,RotationIndex,3,RotationIndex);
   // MIX KEY INTO SCHEDULED MESSAGE
   // W[i] = W[i] XOR ROTR( i mod 31, Key[i mod 8])
   52: D_ROTR(D_ROTR,Inp_KEY[KeyIndex],RotationIndex,IndexedKey)XOR(W[i],IndexedKey,W[i]);
   53: ADD(i,1,i);
   54: LES(i,ROUNDS)JMP(MSGSCHEDULE);
   // ======================================================================================
   // PART 4:  PROCESS SCHEDULE MESSAGE (ROUNDS)
   // ======================================================================================
   // ===================================================
   // STEP4A:  RE-INITIALIZE TEMP BUFFER
   // ===================================================
   55: MOV(0,t);
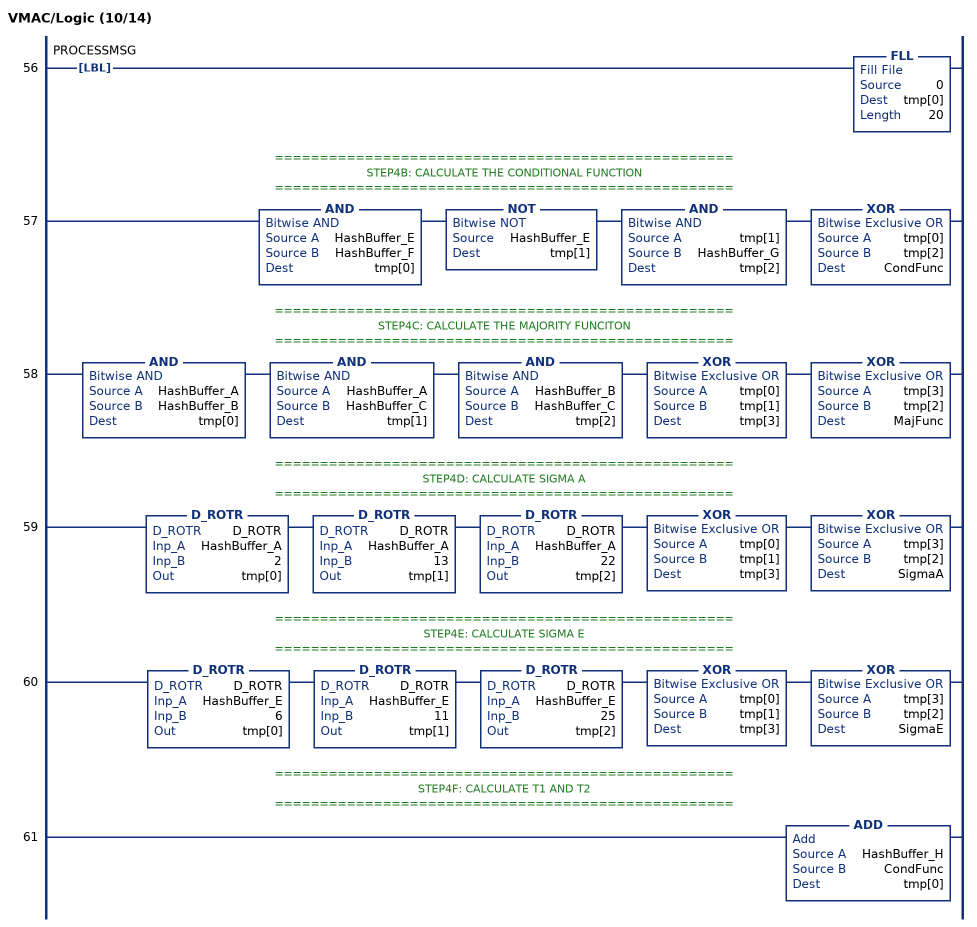
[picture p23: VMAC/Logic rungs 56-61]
   56: LBL(PROCESSMSG)FLL(0,tmp[0],20);
   // ===================================================
   // STEP4B: CALCULATE THE CONDITIONAL FUNCTION
   // ===================================================
   57: AND(HashBuffer_E,HashBuffer_F,tmp[0])NOT(HashBuffer_E,tmp[1])AND(tmp[1],HashBuffer_G,tmp[2])XOR(tmp[0],tmp[2],CondFunc);
   // ===================================================
   // STEP4C: CALCULATE THE MAJORITY FUNCITON
   // ===================================================
   58: AND(HashBuffer_A,HashBuffer_B,tmp[0])AND(HashBuffer_A,HashBuffer_C,tmp[1])AND(HashBuffer_B,HashBuffer_C,tmp[2])XOR(tmp[0],tmp[1],tmp[3])XOR(tmp[3],tmp[2],MajFunc);
   // ===================================================
   // STEP4D: CALCULATE SIGMA A
   // ===================================================
   59: D_ROTR(D_ROTR,HashBuffer_A,2,tmp[0])D_ROTR(D_ROTR,HashBuffer_A,13,tmp[1])D_ROTR(D_ROTR,HashBuffer_A,22,tmp[2])XOR(tmp[0],tmp[1],tmp[3])XOR(tmp[3],tmp[2],SigmaA);
   // ===================================================
   // STEP4E: CALCULATE SIGMA E
   // ===================================================
   60: D_ROTR(D_ROTR,HashBuffer_E,6,tmp[0])D_ROTR(D_ROTR,HashBuffer_E,11,tmp[1])D_ROTR(D_ROTR,HashBuffer_E,25,tmp[2])XOR(tmp[0],tmp[1],tmp[3])XOR(tmp[3],tmp[2],SigmaE);
   // ===================================================
   // STEP4F: CALCULATE T1 AND T2
   // ===================================================
   61: ADD(HashBuffer_H,CondFunc,tmp[0]);
